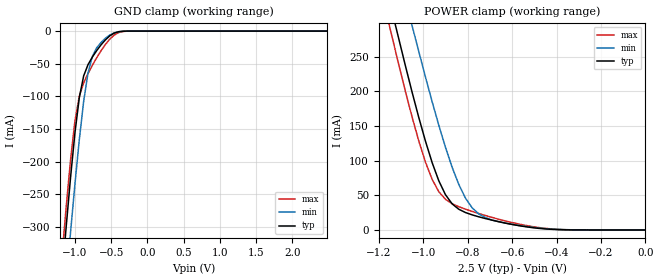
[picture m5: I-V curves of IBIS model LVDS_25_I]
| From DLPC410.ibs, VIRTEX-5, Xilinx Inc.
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|   Model LVDS_25_I
[Model]  LVDS_25_I
Model_type   Input
Polarity   Non-Inverting
Vinl = 1.025
Vinh = 1.375
C_comp   6.0000pF   6.0000pF   6.0000pF
[Model Spec]
Vinl   1.025   0.125   2.025
Vinh   1.375   0.475   2.375
[Temperature Range]   25.0000   85.0000   0.0
[Voltage Range]   2.5000V   2.3750V   2.6250V
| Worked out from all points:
|   GND clamp passes 1 mA (typ) near -0.40 V on its own axis
|   POWER clamp passes 1 mA (typ) near -0.43 V on its own axis
[GND_clamp]
|Voltage   I(typ)   I(min)   I(max)
-2.5V     -2.205A    -2.201A    -2.217A
-1.18V    -378.2mA   -462.1mA   -347.2mA
-1.12V    -298.9mA   -384.1mA   -268.7mA
-1.06V    -223.8mA   -307.7mA   -197mA
-1V       -156.1mA   -234.6mA   -137.9mA
-940mV    -102.2mA   -166.8mA   -99.83mA
-880mV    -68.83mA   -108.2mA   -79.51mA
-820mV    -51.57mA   -64.34mA   -65.27mA
-700mV    -29.96mA   -25.72mA   -40.91mA
-520mV    -7.399mA   -6.106mA   -12.47mA
-280mV    -46.73uA   -67.7uA    -122.5uA
2.48V     11.1nA     564.1nA    20.99nA
[POWER_clamp]
|Voltage   I(typ)   I(min)   I(max)
-2.49V    2.095A     2.089A     2.108A
-1.17V    354.5mA    443.8mA    318.7mA
-1.14V    315mA      406.5mA    278.4mA
-1.11V    275.8mA    369.1mA    238.4mA
-1.05V    198.7mA    294.6mA    162.8mA
-990mV    128.2mA    220.8mA    97.97mA
-960mV    97.28mA    185.2mA    73.02mA
-900mV    50.94mA    119.4mA    44.35mA
-810mV    25.18mA    45.99mA    30.01mA
-750mV    19mA       23.14mA    23.73mA
-480mV    2.327mA    2.844mA    3.493mA
0V        11.82nA    60.98nA    23.86nA
